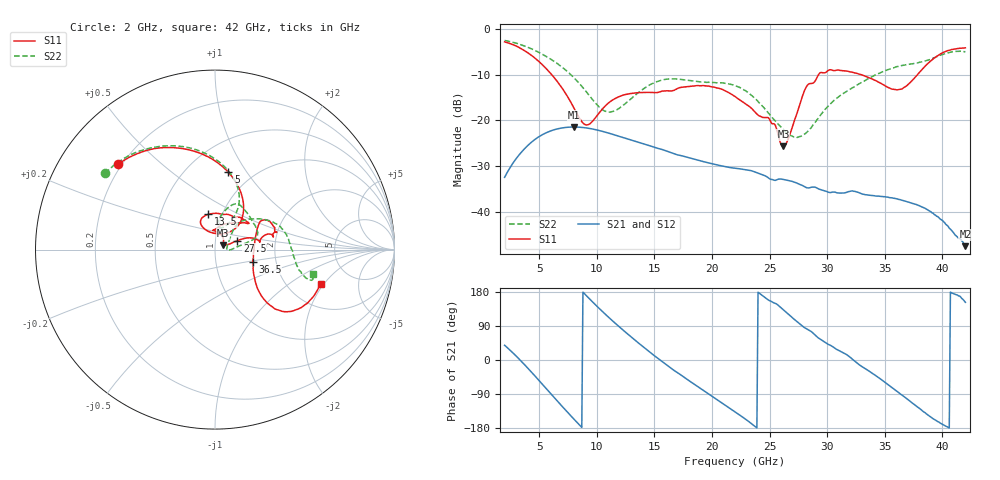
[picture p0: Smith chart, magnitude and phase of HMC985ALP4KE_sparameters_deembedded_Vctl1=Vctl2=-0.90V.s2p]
!s2p File: Measurements: S11, S21, S12, S22
# GHz S dB R 50.0
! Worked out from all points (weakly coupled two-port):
!   401 points, 2 GHz to 42 GHz, reference 50 ohm
!   highest |S21| = -21.45 dB at 8 GHz (marker M1); lowest = -47.5 dB at 42 GHz (marker M2)
!   lowest |S11| = -25.7 dB at 26.2 GHz (marker M3), VSWR 1.11, Z = 54.7 + j2.74 ohm
!   |S11| at or under -10 dB: 6.084 GHz to 29.26 GHz (23.17 GHz wide, 131 % of centre); 32.92 GHz to 37.84 GHz (4.923 GHz wide, 13.9 % of centre)
!   |S22| runs from -23.7 to -2.5 dB; largest |S21 - S12| = 0.00016
!   S11 on the Smith chart (normalised r, x): 2 GHz: 0.18, +0.36; 5 GHz: 0.78, +0.83; 13.5 GHz: 0.86, +0.35; 27.5 GHz: 1.28, +0.13; 36.5 GHz: 1.51, -0.21; 42 GHz: 2.99, -1.87
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2  -2.85 138.8  -32.44 38.9  -32.43 38.9  -2.54 145.3
3.4  -4.28 111.6  -27.12 -1.9  -27.12 -1.9  -3.46 122.6
5  -7.19 80.2  -23.54 -54.5  -23.54 -54.5  -5.18 97.9
6.3  -10.65 57.2  -22.05 -98.9  -22.06 -98.9  -7.12 79.7
8  -17.19 48.4  -21.45 -155.5  -21.45 -155.5  -10.62 62.9
8.7  -20.27 65.0  -21.53 -177.8  -21.54 -177.8  -12.56 60.1
9.4  -20.75 94.7  -21.77 160.4  -21.78 160.4  -14.74 60.8
11  -16.23 119.2  -22.76 113.5  -22.76 113.5  -18.18 77.2
13.5  -13.96 100.6  -24.68 47.8  -24.69 47.8  -14.16 79.5
15.4  -13.82 74.8  -26.18 2.2  -26.18 2.2  -11.38 68.4
18.9  -12.44 38.7  -28.78 -72.9  -28.78 -73.0  -11.56 41.1
22  -14.78 54.7  -30.44 -136.5  -30.46 -136.5  -12.41 16.7
24.9  -19.43 92.1  -32.55 158.2  -32.55 158.2  -18.39 6.5
26.2  -25.69 28.7  -32.91 132.1  -32.91 132.1  -22.04 -2.3
27.5  -17.52 21.6  -33.86 98.2  -33.85 98.0  -23.62 4.8
28.7  -11.91 9.8  -34.58 73.1  -34.60 72.9  -21.28 28.8
31  -9.02 20.6  -35.87 25.2  -35.90 25.1  -14.82 49.0
33.3  -10.33 31.9  -36.23 -22.7  -36.24 -22.6  -11.29 38.8
35.4  -12.91 10.8  -36.88 -67.6  -36.84 -67.5  -8.82 24.2
36.5  -13.12 -17.7  -37.45 -92.6  -37.48 -92.7  -8.00 15.6
39.6  -5.87 -42.6  -41.02 -162.5  -41.02 -163.0  -6.02 -15.4
42  -4.16 -18.1  -47.48 152.3  -47.56 151.9  -4.99 -13.7
